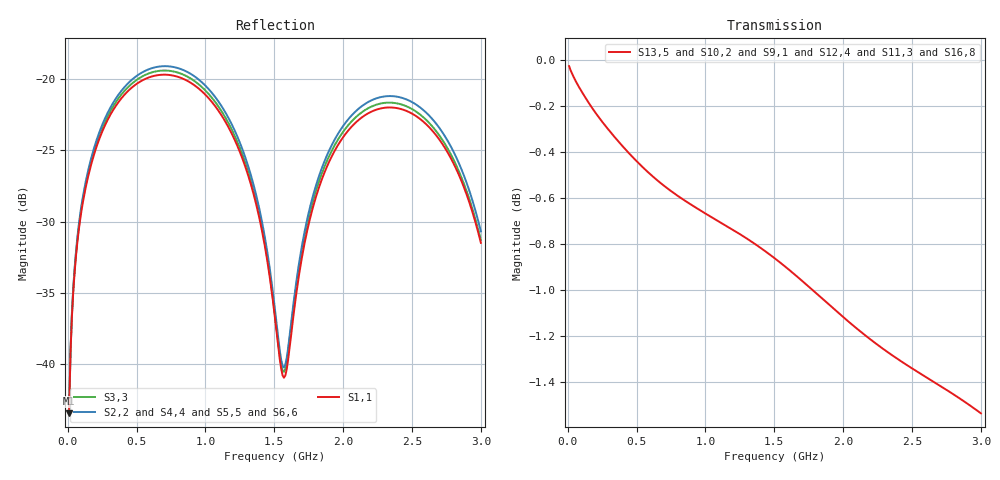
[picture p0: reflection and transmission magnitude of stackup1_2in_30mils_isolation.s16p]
! Touchstone file from project
# GHZ S RI R 50.000000
! Modal data exported
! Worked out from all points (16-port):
!   300 points, 10 MHz to 3 GHz, reference 50 ohm
!   strongest paths, dB at 10 MHz, 760 MHz, 1.51 GHz, 2.26 GHz, 3 GHz:
!     S13,5: 0.0, -0.6, -0.9, -1.2, -1.5
!     S10,2: 0.0, -0.6, -0.9, -1.2, -1.5
!     S9,1: 0.0, -0.6, -0.9, -1.2, -1.5
!     S12,4: 0.0, -0.6, -0.9, -1.2, -1.5
!     S11,3: 0.0, -0.6, -0.9, -1.2, -1.5
!     S16,8: 0.0, -0.6, -0.9, -1.2, -1.5
!   lowest |S11| = -43.4 dB at 10 MHz (marker M1), VSWR 1.01, Z = 50.3 + j0.6 ohm
!   |S11| at or under -10 dB: start of sweep to end of sweep
